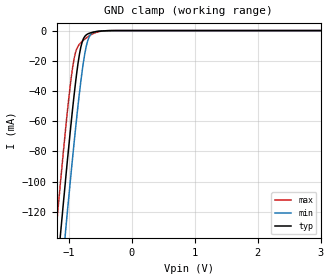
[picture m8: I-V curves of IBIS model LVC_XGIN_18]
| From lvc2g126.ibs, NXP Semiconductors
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|   Model LVC_XGIN_18
[Model]   LVC_XGIN_18
Model_type   Input
Vinl =   0.63V
Vinh =   1.17V
C_comp   3.07pF   2.35pF   3.88pF
[Model Spec]
| Note: The input and output voltage ratings may be exceeded if the input and
|   output current ratings are observed (please refer to the data sheet)
|   Subparameter   typ   min   max
| Thresholds
Vinh   1.17   1.0725   1.2675
Vinl   0.63   0.5775   0.6825
| Overshoot
S_overshoot_high   6.5   6.5   6.5   | Static overshoot
S_overshoot_low   -0.5   -0.5   -0.5
D_overshoot_high   7.2   7.2   7.2   | Dynamic overshoot
D_overshoot_low   -0.95   -0.9   -1.0
D_overshoot_time   3n   3n   3n
|Ambient temperature:   25   85   -40
[Temperature Range]   25   85   -40
[Voltage Range]   1.80V   1.65V   1.95V
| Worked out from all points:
|   GND clamp passes 1 mA (typ) near -0.61 V on its own axis
|Process Range   nominal   slow   fast
[GND_clamp]
| voltage   I(typ)   I(min)   I(max)
-5.5V     -2.277A    -2.307A    -2.246A
-1.221V   -173.6mA   -208.2mA   -138.8mA
-1.2V     -163.7mA   -198.3mA   -129mA
-1.136V   -134.3mA   -168.7mA   -99.82mA
-1.071V   -105.4mA   -139.6mA   -71.73mA
-1.05V    -95.98mA   -130mA     -62.73mA
-942.9mV  -51.21mA   -83.48mA   -24.05mA
-900mV    -35.22mA   -65.87mA   -14.8mA
-835.7mV  -15.71mA   -41.31mA   -9.021mA
-728.6mV  -2.901mA   -10.64mA   -4.899mA
-642.9mV  -1.321mA   -1.88mA    -2.576mA
5.5V      0A         0A         0A
